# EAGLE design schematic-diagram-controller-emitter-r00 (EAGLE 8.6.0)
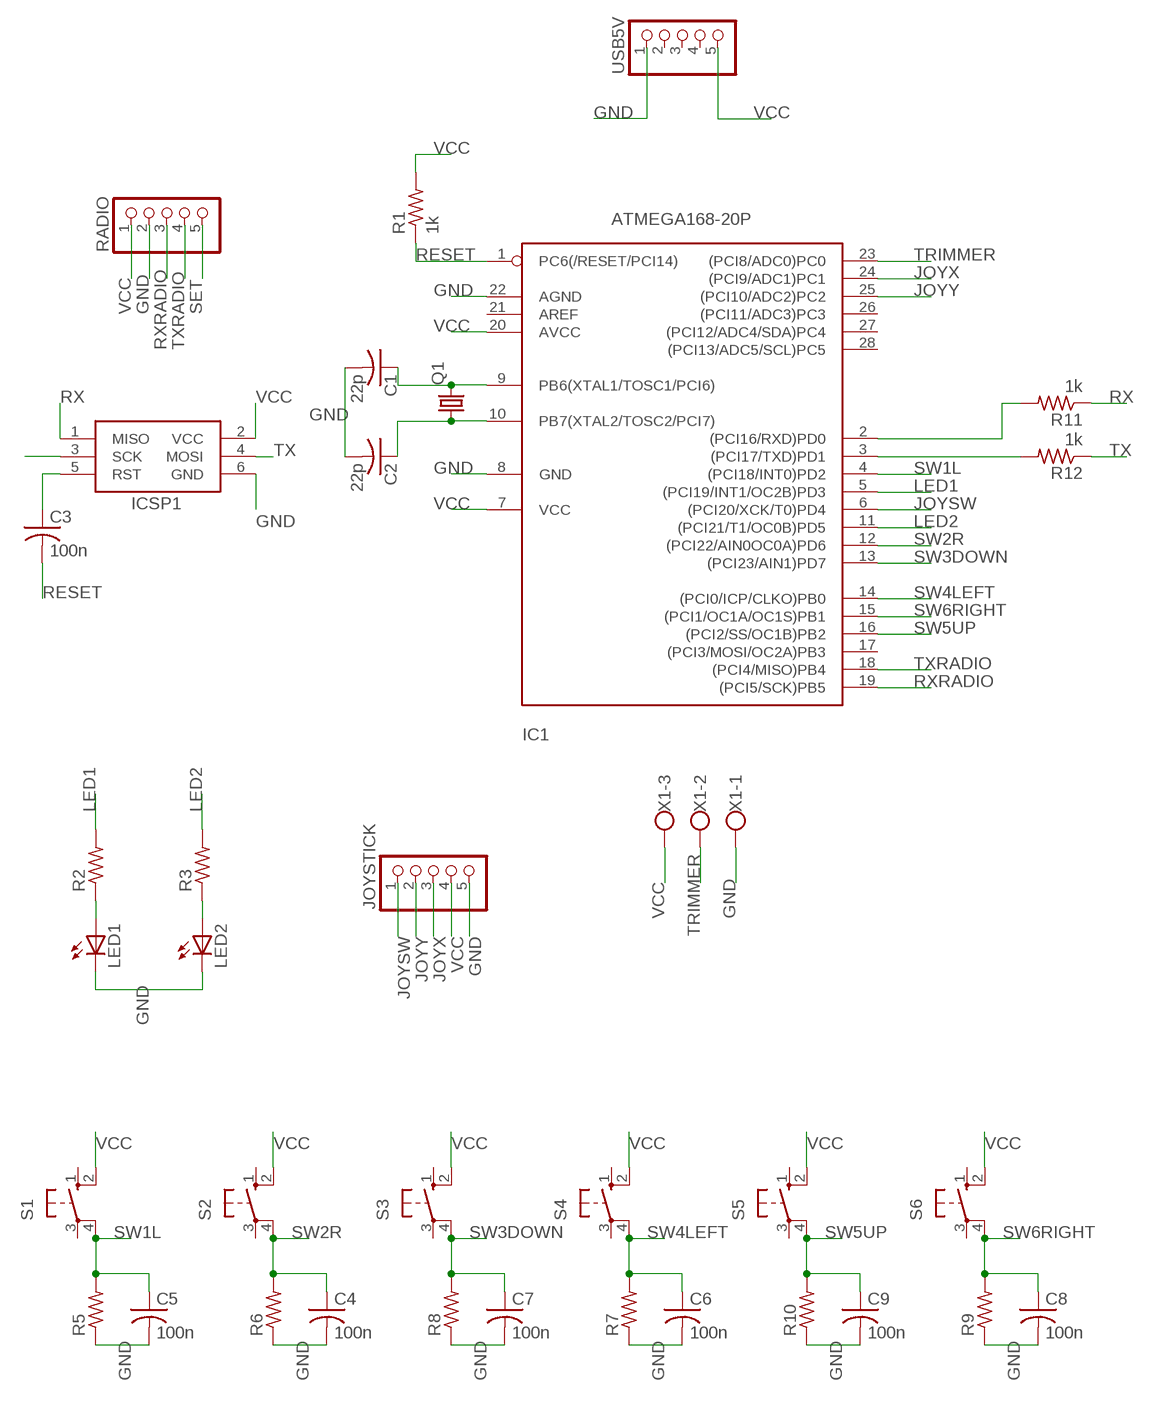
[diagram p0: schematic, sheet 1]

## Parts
C1  22p  C-US025-025X050  [C025-025X050]
C2  22p  C-US025-025X050  [C025-025X050]
C3  100n  C-US025-025X050  [C025-025X050]
C4  100n  C-US025-025X050  [C025-025X050]
C5  100n  C-US025-025X050  [C025-025X050]
C6  100n  C-US025-025X050  [C025-025X050]
C7  100n  C-US025-025X050  [C025-025X050]
C8  100n  C-US025-025X050  [C025-025X050]
C9  100n  C-US025-025X050  [C025-025X050]
IC1  ATMEGA168-20P  [DIL28-3]
ICSP1  AVRISP-6  [AVRISP]
JOYSTICK  PINHD-1X5  [1X05]
LED1  LED5MM  [LED5MM]
LED2  LED5MM  [LED5MM]
Q1  CRYSTALHC49S  [HC49/S]
R1  1k  R-US_0207/12  [0207/12]
R2  R-US_0207/12  [0207/12]
R3  R-US_0207/12  [0207/12]
R5  R-US_0207/12  [0207/12]
R6  R-US_0207/12  [0207/12]
R7  R-US_0207/12  [0207/12]
R8  R-US_0207/12  [0207/12]
R9  R-US_0207/12  [0207/12]
R10  R-US_0207/12  [0207/12]
R11  1k  R-US_0207/12  [0207/12]
R12  1k  R-US_0207/12  [0207/12]
RADIO  PINHD-1X5  [1X05]
S1  10-XX  [B3F-10XX]
S2  10-XX  [B3F-10XX]
S3  40-XX-ROUND  [B3F-40XX-ROUND]
S4  40-XX-ROUND  [B3F-40XX-ROUND]
S5  40-XX-ROUND  [B3F-40XX-ROUND]
S6  40-XX-ROUND  [B3F-40XX-ROUND]
USB5V  PINHD-1X5  [1X05]
X1  W237-103  [W237-103]

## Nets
DTR: C3.1 ICSP1.5(RST)
GND: C1.2 C2.2 C4.2 C5.2 C6.2 C7.2 C8.2 C9.2 IC1.8(GND) IC1.22(AGND) ICSP1.6(GND) JOYSTICK.5 LED1.K(C) LED2.K(C) R5.1 R6.1 R7.1 R8.1 R9.1 R10.1 RADIO.2 USB5V.1 X1.1
JOYSW: IC1.6((PCI20/XCK/T0)PD4) JOYSTICK.1
JOYX: IC1.24((PCI9/ADC1)PC1) JOYSTICK.3
JOYY: IC1.25((PCI10/ADC2)PC2) JOYSTICK.2
LED1: IC1.5((PCI19/INT1/OC2B)PD3) R2.2
LED2: IC1.11((PCI21/T1/OC0B)PD5) R3.2
N$1: LED2.A R3.1
N$2: C1.1 IC1.9(PB6(XTAL1/TOSC1/PCI6)) Q1.2
N$3: C2.1 IC1.10(PB7(XTAL2/TOSC2/PCI7)) Q1.1
N$4: LED1.A R2.1
N$5: IC1.2((PCI16/RXD)PD0) R11.2
N$6: IC1.3((PCI17/TXD)PD1) R12.2
N$8: ICSP1.3(SCK)
RESET: C3.2 IC1.1(PC6(/RESET/PCI14)) R1.1
RX: ICSP1.1(MISO) R11.1
RXRADIO: IC1.19((PCI5/SCK)PB5) RADIO.3
SET: RADIO.5
SW1L: C5.1 IC1.4((PCI18/INT0)PD2) R5.2 S1.4(P1)
SW2R: C4.1 IC1.12((PCI22/AIN0OC0A)PD6) R6.2 S2.4(P1)
SW3DOWN: C7.1 IC1.13((PCI23/AIN1)PD7) R8.2 S3.4(P1)
SW4LEFT: C6.1 IC1.14((PCI0/ICP/CLKO)PB0) R7.2 S4.4(P1)
SW5UP: C9.1 IC1.16((PCI2/SS/OC1B)PB2) R10.2 S5.4(P1)
SW6RIGHT: C8.1 IC1.15((PCI1/OC1A/OC1S)PB1) R9.2 S6.4(P1)
TRIMMER: IC1.23((PCI8/ADC0)PC0) X1.2
TX: ICSP1.4(MOSI) R12.1
TXRADIO: IC1.18((PCI4/MISO)PB4) RADIO.4
VCC: IC1.7(VCC) IC1.20(AVCC) ICSP1.2(VCC) JOYSTICK.4 R1.2 RADIO.1 S1.2(S1) S2.2(S1) S3.2(S1) S4.2(S1) S5.2(S1) S6.2(S1) USB5V.5 X1.3
Unconnected: IC1.17((PCI3/MOSI/OC2A)PB3) IC1.21(AREF) IC1.26((PCI11/ADC3)PC3) IC1.27((PCI12/ADC4/SDA)PC4) IC1.28((PCI13/ADC5/SCL)PC5) S1.1(S) S1.3(P) S2.1(S) S2.3(P) S3.1(S) S3.3(P) S4.1(S) S4.3(P) S5.1(S) S5.3(P) S6.1(S) S6.3(P) USB5V.2 USB5V.3 USB5V.4

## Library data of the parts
C1-C9 = adafruit:C-US: CAPACITOR, American symbol
IC1 = adafruit:ATMEGA168*P: MICROCONTROLLER 16 kBytes FLASH 1 kBytes SRAM 512 Bytes EEPROM USART 8-channel 10 bit ADC
ICSP1 = adafruit:AVRISP: AVR ISP HEADER Standard 6 pin header for AVR programming
JOYSTICK RADIO USB5V = pinhead:PINHD-1X5: PIN HEADER
LED1 LED2 = adafruit:LED: LED
Q1 = adafruit:CRYSTAL: CRYSTAL; OC_FARNELL: 1667008; OC_NEWARK: unknown
R1-R3 R5-R12 = adafruit:R-US_: RESISTOR, American symbol
S1 S2 = switch-omron:10-XX: OMRON SWITCH; MPN: B3F-1000; OC_FARNELL: 176432; OC_NEWARK: 36M3542
S3-S6 = adafruit:40-XX: OMRON SWITCH
X1 = con-wago-500:W237-103: WAGO SCREW CLAMP; MPN: 237-103; OC_FARNELL: unknown; OC_NEWARK: 18M7116

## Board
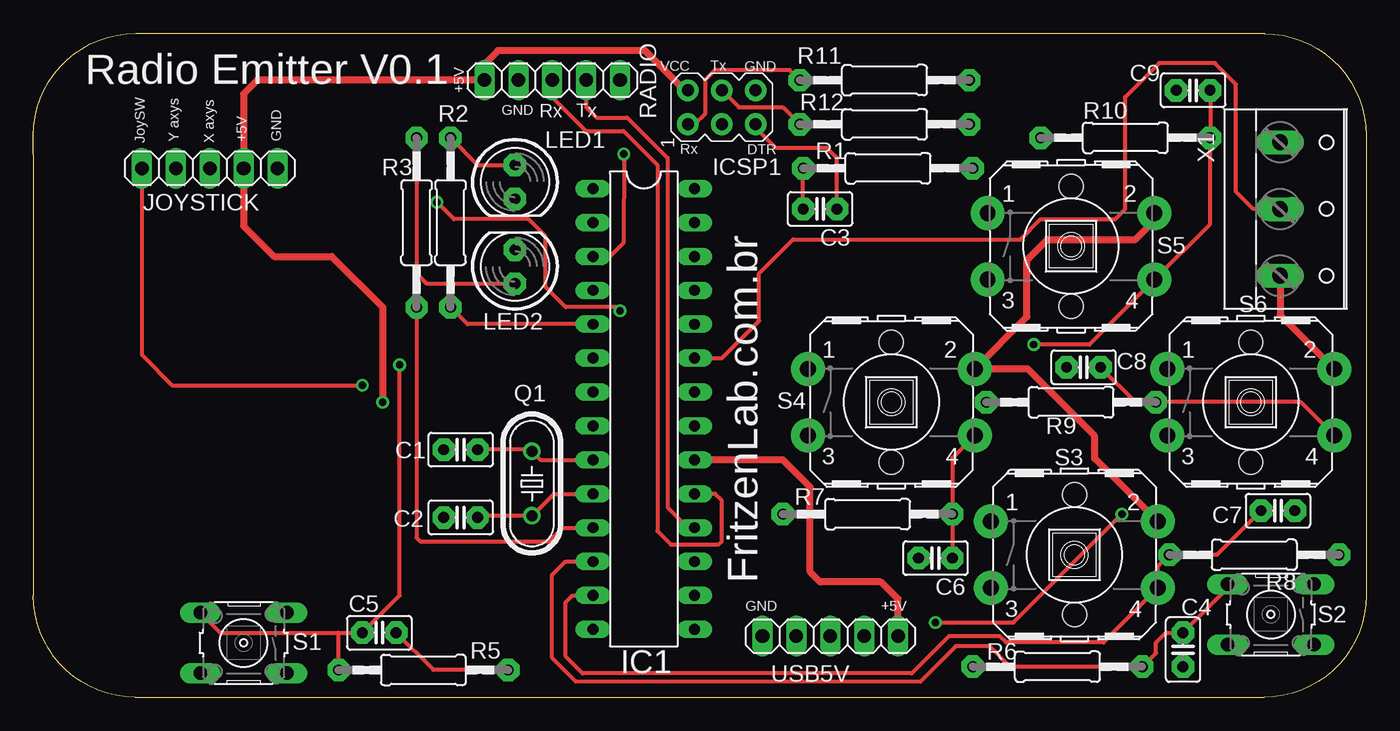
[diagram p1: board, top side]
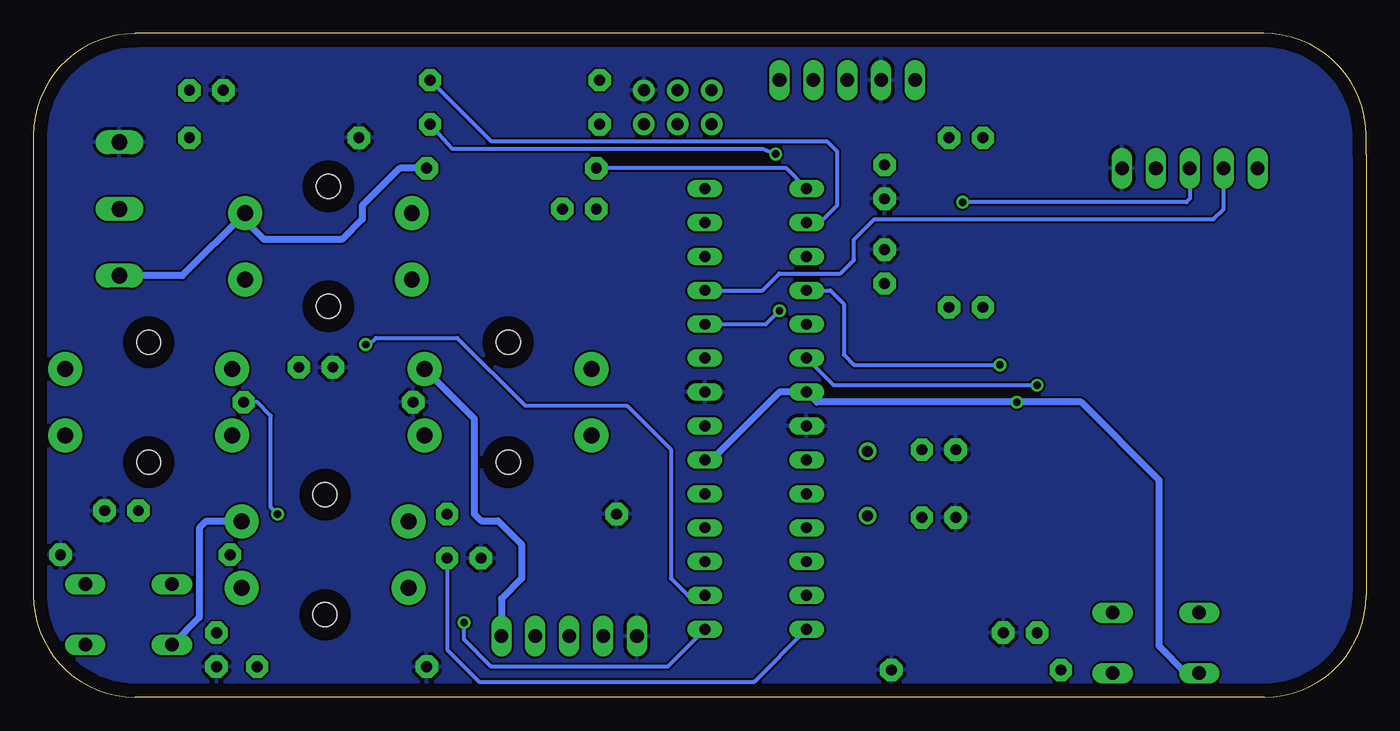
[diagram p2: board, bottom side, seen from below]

Size 99.82 x 49.73 mm. Coordinates in mm from the lower left corner, seen from the top.
Outline: 0,42.09 0,40.64 0,7.62 arc90 7.62,0 92.2,0 arc90 99.82,7.62 99.82,42.09 arc90 92.2,49.71 arc90 92.18,49.73 7.7,49.73
Outline: 0,42.09 0,42.16
Outline: 0,42.09 arc-90 7.7,49.73
Outline: 7.67,49.73 7.7,49.73
Copper layers (1*16): Top 0.035mm / dielectric 1.5mm / Bottom 0.035mm
Design rules "default": minimum track width 6mil, minimum drill 0.35mm, track to track 6mil, track to pad 6mil, pad to pad 6mil, via to via 6mil, smd to smd 6mil, copper to edge 40mil, drill to drill 6mil, minimum pad ring 10mil, minimum via ring 8mil, stop-mask expansion 4mil, vias tented up to drill 0mil, thermal gap 10mil

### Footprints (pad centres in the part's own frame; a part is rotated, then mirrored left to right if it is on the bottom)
C025-025X050 = drill 0.813 pad 1.676 octagon: 1 -1.27,0; 2 1.27,0
DIL28-3 = drill 0.813 long: 1 -16.51,-3.81; 2 -13.97,-3.81; 3 -11.43,-3.81; 4 -8.89,-3.81; 5 -6.35,-3.81; 6 -3.81,-3.81; 7 -1.27,-3.81; 8 1.27,-3.81; 9 3.81,-3.81; 10 6.35,-3.81; 11 8.89,-3.81; 12 11.43,-3.81; 13 13.97,-3.81; 14 16.51,-3.81; 15 16.51,3.81; 16 13.97,3.81; 17 11.43,3.81; 18 8.89,3.81; 19 6.35,3.81; 20 3.81,3.81; 21 1.27,3.81; 22 -1.27,3.81; 23 -3.81,3.81; 24 -6.35,3.81; 25 -8.89,3.81; 26 -11.43,3.81; 27 -13.97,3.81; 28 -16.51,3.81
AVRISP = drill 0.9 pad 1.626: 1 -1.27,2.54; 2 1.27,2.54; 3 -1.27,0; 4 1.27,0; 5 -1.27,-2.54; 6 1.27,-2.54
1X05 = drill 1.016 long: 1 -5.08,0; 2 -2.54,0; 3 0,0; 4 2.54,0; 5 5.08,0
LED5MM = drill 0.813 pad 1.676 octagon: A -1.27,0; K 1.27,0
HC49/S = drill 0.813: 1 -2.413,0; 2 2.413,0
0207/12 = drill 0.813 pad 1.676 octagon: 1 -6.35,0; 2 6.35,0
B3F-10XX = drill 1.016 long: 1 -3.251,2.261; 2 3.251,2.261; 3 -3.251,-2.261; 4 3.251,-2.261
B3F-40XX-ROUND = drill 1.194 pad 2.54: 1 -6.248,2.489; 2 6.248,2.489; 3 -6.248,-2.489; 4 6.248,-2.489 | hole 1.803: 0,-4.496; 0,4.496
W237-103 = drill 1.194 long: 1 -5,-1.29; 2 0,-1.29; 3 5,-1.29

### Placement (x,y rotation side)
C1  32,18.54 180 top
C2  32,13.46 180 top
C3  58.93,36.58 180 top
C4  86.11,3.56 270 top
C5  25.91,4.83 0 top
C6  67.56,10.41 180 top
C7  93.22,13.97 0 top
C8  78.66,24.71 180 top
C9  86.87,45.47 180 top
IC1  45.72,21.59 270 top
ICSP1  51.56,44.2 90 top
JOYSTICK  13.21,39.62 0 top
LED1  36.07,38.61 270 top
LED2  36.07,32.26 90 top
Q1  37.34,16 90 top
R1  64.01,39.62 0 top
R2  31.24,35.56 270 top
R3  28.7,35.56 270 top
R5  29.21,2.03 180 top
R6  76.71,2.29 0 top
R7  62.48,13.72 0 top
R8  91.44,10.67 180 top
R9  77.72,22.1 0 top
R10  81.79,41.91 0 top
R11  63.75,46.23 0 top
R12  63.75,42.93 0 top
RADIO  38.86,46.23 0 top
S1  15.75,4.06 180 top
S2  92.68,6.2 180 top
S3  77.98,10.67 0 top
S4  64.26,22.1 0 top
S5  77.72,33.78 0 top
S6  91.19,22.1 0 top
USB5V  59.69,4.57 0 top
X1  94.67,36.58 270 top

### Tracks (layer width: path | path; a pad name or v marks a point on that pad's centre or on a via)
DTR
  Top 0.305: C3.1 60.2,40.39 59.44,41.15 55.63,41.15 54.1,42.67 ICSP1.5
GND
  Top 0.305: R5.1 29.97,2.03 C5.2
  pour Bottom: 0.99,0.2 100.08,0.2 100.08,0.41 100.08,50.29 0.2,50.29 0.2,0.2
JOYSW  (via drill 0.55)
  Top 0.305: JOYSTICK.1 8.13,25.65 10.41,23.37 v24.64,23.37
  Bottom 0.305: v24.64,23.37 39.88,23.37 IC1.6
JOYX  (via drill 0.55)
  Top 0.305: v43.94,28.96 43.69,29.21 39.88,29.21 38.35,30.73 38.35,34.54 37.08,35.81 31.5,35.81 v30.23,37.08
  Bottom 0.305: IC1.24 44.96,27.94 v43.94,28.96 | JOYSTICK.3 13.21,37.34 13.46,37.08 v30.23,37.08
JOYY
  Bottom 0.305: IC1.25 45.21,30.48 43.94,31.75 39.37,31.75 38.35,32.77 38.35,34.29 36.83,35.81 11.43,35.81 10.67,36.58 JOYSTICK.2
LED1
  Top 0.305: IC1.5 32.51,27.94 R2.2
LED2
  Top 0.305: 41.66,12.7 IC1.11 39.62,12.7 38.61,11.68 28.96,11.68 28.7,11.94 R3.2
N$1
  Top 0.305: R3.1 28.7,31.75 29.46,30.99 LED2.A
N$2
  Top 0.305: IC1.9 37.97,17.78 Q1.2 37.21,18.54 C1.1
N$3
  Top 0.305: IC1.10 38.99,15.24 Q1.1 33.4,13.59 C2.1
N$4
  Top 0.305: R2.1 33.27,39.88 LED1.A
N$5
  Bottom 0.305: R11.2 65.53,41.66 40.39,41.66 39.62,40.89 39.62,36.83 40.89,35.56 IC1.2
N$6  (via drill 0.55)
  Top 0.305: IC1.3 43.18,33.02 44.2,34.04 v44.22,40.69
  Bottom 0.305: v44.22,40.69 45.21,41.07 68.43,41.07 R12.2
RESET
  Top 0.305: C3.2 R1.1
  Bottom 0.305: IC1.1 43.43,39.62 R1.1
RX
  Top 0.305: R11.1 56.64,46.99 51.05,46.99 50.29,46.23 50.29,43.69 49.53,42.93 ICSP1.1
RXRADIO
  Top 0.305: RADIO.3 38.86,44.96 41.4,42.42 44.2,42.42 46.74,39.88 46.74,12.45 47.75,11.43 51.31,11.43 51.56,11.68 51.56,14.73 51.05,15.24 IC1.19
SW1L  (via drill 0.55)
  Top 0.305: S1.4 13.99,4.83 22.86,4.83 | 22.86,4.83 C5.1 27.43,7.62 v27.43,24.89 | R5.2 22.86,4.83
  Bottom 0.305: v27.43,24.89 38.35,24.89 39.12,25.65 39.12,29.46 40.13,30.48 IC1.4
SW2R
  Top 0.305: IC1.12 39.88,10.16 38.86,9.14 38.86,2.95 40.64,1.17 66.45,1.17 69.09,3.81 71.63,3.81 73.15,2.29 R6.2 84.07,3.3 84.07,4.06 84.84,4.83 C4.1 89.43,8.15 S2.4
SW3DOWN
  Top 0.305: C7.1 88.65,10.67 R8.2 84.23,9.8 S3.4 80.15,4.1 72.86,4.1 72.39,4.57 68.58,4.57 65.79,1.78 41.15,1.78 39.88,3.05 39.88,7.11 40.39,7.62 IC1.13
SW4LEFT
  Top 0.305: S4.4 68.83,17.93 R7.2 C6.1
  Bottom 0.305: C6.1 68.83,3.56 66.45,1.17 45.82,1.17 IC1.14
SW5UP  (via drill 0.55)
  Top 0.305: C9.1 R10.2 88.14,35.46 S5.4 79.1,26.42 v74.93,26.42
  Bottom 0.305: v74.93,26.42 74.68,26.42 74.17,26.92 68.07,26.92 62.99,21.84 55.37,21.84 52.07,18.54 52.07,8.89 50.8,7.62 IC1.16
SW6RIGHT  (via drill 0.55)
  Top 0.305: S6.4 94.94,22.1 R9.2 82.55,22.1 C8.1 | v67.56,5.59 73.41,5.59 v81.53,13.72
  Bottom 0.305: IC1.15 52.32,2.29 65.53,2.29 67.56,4.32 v67.56,5.59 | v81.53,13.72 82.04,14.22 82.04,21.08 83.06,22.1 R9.2
TRIMMER
  Top 0.305: IC1.23 51.56,25.4 54.36,28.19 54.36,31.75 56.9,34.29 73.91,34.29 75.44,35.81 81.03,35.81 81.79,36.58 81.79,44.96 84.33,47.5 88.49,47.5 90.07,45.92 90.07,37.87 91.36,36.58 X1.2
TX
  Top 0.305: ICSP1.4 52.83,44.2 56.13,44.2 R12.1
TXRADIO
  Top 0.305: RADIO.4 41.4,44.2 42.16,43.43 44.45,43.43 47.5,40.39 47.5,14.22 49.02,12.7 IC1.18
VCC  (via drill 0.55)
  Top 0.508: ICSP1.2 48.77,45.47 45.8,48.44 34.8,48.44 33.78,47.42 RADIO.1 16.76,46.23 15.75,45.21 JOYSTICK.4 15.75,35.31 18.03,33.02 22.35,33.02 26.16,29.21 v26.16,22.1 | IC1.20 56.13,17.78 58.17,15.75 58.17,9.4 58.93,8.64 63.5,8.64 64.77,7.37 USB5V.5 | S5.2 83.97,35.71 82.55,34.29 75.95,34.29 74.42,32.77 74.42,28.5 S4.2 74.47,24.59 79.5,19.56 79.5,17.88 S3.2 | X1.3 93.38,28.65 S6.2
  Bottom 0.508: IC1.20 49.02,17.78 43.94,22.86 IC1.7 41.15,22.1 v26.16,22.1 21.34,22.1 15.49,16.26 15.49,3.81 13.49,1.8 S1.2 | S3.2 86.92,13.16 87.4,12.68 87.4,5.97 S2.2 | 84.35,35.89 84.25,35.99 | 84.25,35.99 S5.2 88.67,31.58 X1.3 | S4.2 66.8,20.88 66.8,13.72 66.29,13.21 65.02,13.21 63.25,11.43 63.25,8.89 64.77,7.37 USB5V.5 | R1.2 72.39,39.62 75.18,36.83 75.18,35.81 76.71,34.29 82.55,34.29 84.25,35.99

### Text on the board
tNames: Radio Emitter V0.1 | VCC | Tx | GND | X axys | +5V | +5V | GND | GND | Rx | Tx | JoySW | Y axys | Rx | DTR | FritzenLab.com.br | GND | +5V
